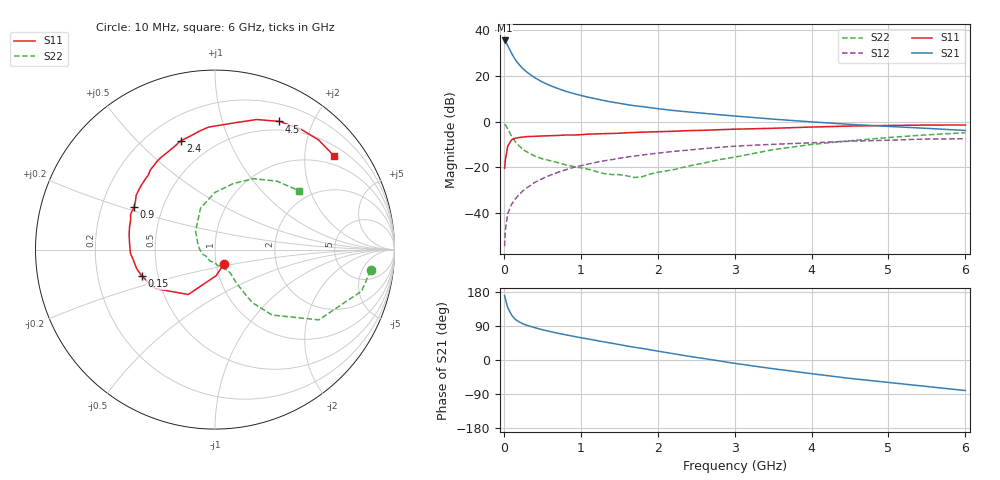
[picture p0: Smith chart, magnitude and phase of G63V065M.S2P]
! SIEMENS Small Signal Semiconductors
! BFG193
! Si NPN RF Bipolar Junction Transistor in SOT223
! VCE = 3 V  IC = 65 mA
! Common Emitter S-Parameters:  August  1996
# GHz  S  MA  R  50
!  f  S11  S21  S12  S22
! GHz  MAG  ANG  MAG  ANG  MAG  ANG  MAG  ANG
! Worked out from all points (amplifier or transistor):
!   36 points, 10 MHz to 6 GHz, reference 50 ohm
!   highest |S21| = 35.5 dB at 10 MHz (marker M1)
!   |S21| within 3 dB of that: start of sweep to 61.99 MHz
!   unconditionally stable (mu >= 1): start of sweep to 10.27 MHz; 324.5 MHz to 2.419 GHz
!   at 250 MHz: K = 0.97, MSG = 26.6 dB, |S12| = -30.2 dB
!   at 1.4 GHz: K = 1.06, MAG = 11.1 dB, |S12| = -16.6 dB
!   at 6 GHz: K = 0.92, MSG = 1.8 dB, |S12| = -7.5 dB
!   S11 on the Smith chart (normalised r, x): 10 MHz: 1.08, -0.18; 150 MHz: 0.40, -0.15; 900 MHz: 0.34, +0.22; 2.4 GHz: 0.33, +0.68; 4.5 GHz: 0.39, +1.55; 6 GHz: 0.74, +2.70
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0.01  0.0957 -60.1  59.31 170.0  0.0019 84.0  0.8746 -7.6
0.02  0.1458 -87.6  56.54 161.2  0.0042 78.7  0.8491 -15.8
0.05  0.2912 -120.8  46.1 138.8  0.0097 70.8  0.6985 -34.1
0.1  0.3976 -146.9  31.22 118.8  0.0156 66.2  0.4837 -48.9
0.15  0.4345 -160.4  22.5 107.0  0.0206 67.3  0.3612 -54.9
0.2  0.4494 -166.6  17.55 100.6  0.0256 68.7  0.2943 -56.0
0.25  0.4599 -173.2  14.26 95.4  0.0309 69.7  0.2451 -56.8
0.3  0.4713 -177.3  12.04 91.5  0.0358 70.7  0.2182 -57.4
0.4  0.4771 176.0  9.146 85.6  0.0468 70.4  0.1774 -57.0
0.5  0.4859 169.9  7.333 79.9  0.0566 69.3  0.1541 -56.9
0.6  0.4922 165.4  6.159 75.3  0.0675 68.3  0.1403 -58.5
0.7  0.4982 160.8  5.296 70.8  0.0776 66.8  0.1276 -61.6
0.9  0.509 152.4  4.138 62.7  0.0992 63.0  0.1046 -66.7
1.1  0.5329 145.6  3.402 55.3  0.1185 59.4  0.091 -79.0
1.3  0.5455 138.5  2.891 47.9  0.1392 55.2  0.0732 -92.0
1.6  0.5716 129.0  2.356 36.8  0.168 48.2  0.0653 -122.8
2.2  0.6151 112.0  1.754 16.8  0.2227 34.4  0.0884 175.3
2.4  0.6355 107.5  1.626 10.0  0.2393 30.1  0.1068 156.4
3.5  0.7148 81.2  1.133 -23.0  0.3198 2.5  0.244 109.3
4.5  0.7993 63.3  0.871 -48.6  0.3738 -17.6  0.3815 74.6
5.5  0.8404 46.6  0.712 -69.9  0.4176 -41.1  0.5143 47.9
6  0.8439 38.3  0.641 -80.6  0.4214 -54.5  0.5713 35.0
